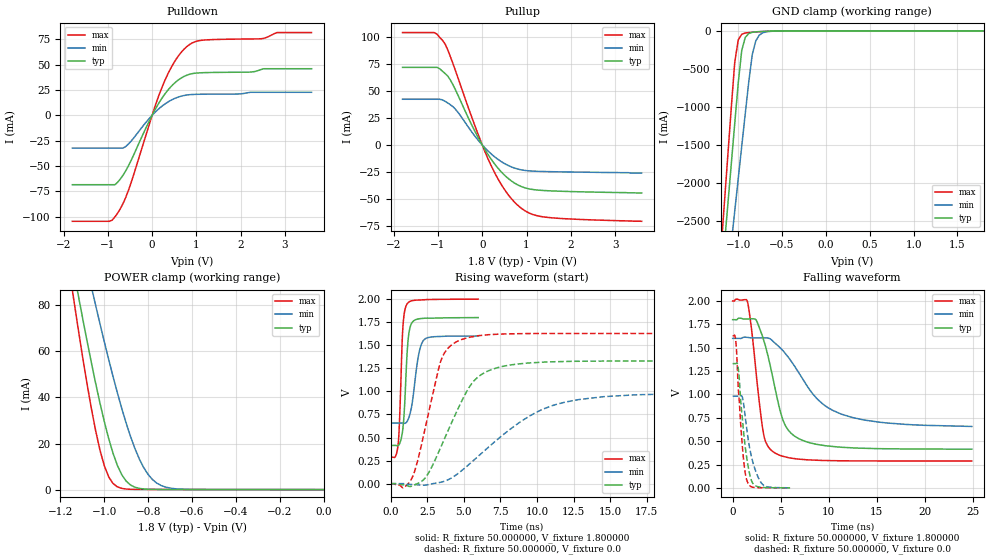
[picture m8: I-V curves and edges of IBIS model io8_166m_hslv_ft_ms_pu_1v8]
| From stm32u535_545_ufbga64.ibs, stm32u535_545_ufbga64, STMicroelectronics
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|   Model io8_166m_hslv_ft_ms_pu_1v8
[Model]  io8_166m_hslv_ft_ms_pu_1v8
Model_type I/O
Polarity   Non-Inverting
Enable   Active-Low
Vinl =   0.540000V
Vinh =   1.260000V
Vmeas =  0.900000V
Cref =   50.000000pF
Rref =   100.000000M
Vref =   0.0V
C_comp   3.358400pF   3.352800pF   3.400400pF
[Temperature Range]   25.000000   0.140000k   -40.000000
[Pullup Reference]   1.800000V   1.600000V   2.000000V
[Pulldown Reference]   0.0V   0.0V   0.0V
[POWER Clamp Reference]   1.800000V   1.600000V   2.000000V
[GND Clamp Reference]   0.0V   0.0V   0.0V
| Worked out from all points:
|   slope of the pulldown table from 0 to 0.27 V, typ, clamps not added: 13.6 ohm
|   slope of the pullup table from 0 to 0.27 V, typ, clamps not added: 15.9 ohm
|   GND clamp passes 1 mA (typ) near -0.51 V on its own axis
|   POWER clamp passes 1 mA (typ) near -0.86 V on its own axis
|   rising waveform, R_fixture 50.000000, V_fixture 1.800000: 20-80 % time 283ps typ, 490ps min, 231ps max; typ from 0.414 V to 1.8 V
|   rising waveform, R_fixture 50.000000, V_fixture 0.0: 20-80 % time 2.38ns typ, 4.83ns min, 1.41ns max; typ from 0 V to 1.33 V
|   falling waveform, R_fixture 50.000000, V_fixture 1.800000: 20-80 % time 1.98ns typ, 4.45ns min, 1.12ns max; typ from 1.8 V to 0.414 V
|   falling waveform, R_fixture 50.000000, V_fixture 0.0: 20-80 % time 798ps typ, 1.05ns min, 633ps max; typ from 1.33 V to 0 V
[Pulldown]
|Voltage   I(typ)   I(min)   I(max)
-1.8V     -68.38mA   -32.32mA   -104.4mA
-960mV    -68.38mA   -32.32mA   -104.4mA
-780mV    -66.08mA   -32.32mA   -96.43mA
-540mV    -50.22mA   -28.51mA   -74.66mA
0V        0A         0A         0A
240mV     18.04mA    9.6mA      29.42mA
480mV     30.68mA    16.02mA    50.95mA
780mV     39.48mA    19.99mA    67.56mA
1.14V     41.99mA    20.78mA    74.01mA
2.46V     45.1mA     22.69mA    75.45mA
2.82V     45.89mA    22.69mA    81.54mA
3.6V      45.89mA    22.69mA    81.54mA
[Pullup]
|Voltage   I(typ)   I(min)   I(max)
-1.8V     71.66mA    42.2mA     103.8mA
-1.08V    71.66mA    42.2mA     103.8mA
-840mV    66.03mA    40.35mA    93.39mA
-720mV    60mA       37.16mA    81.6mA
-600mV    50.51mA    32.72mA    68.08mA
-180mV    13.77mA    8.913mA    19.32mA
180mV     -11.9mA    -7.442mA   -17.26mA
480mV     -26.98mA   -16.65mA   -39.76mA
840mV     -37.65mA   -22.63mA   -57.07mA
1.08V     -40.74mA   -24.01mA   -63.22mA
1.44V     -42.19mA   -24.58mA   -66.73mA
3.6V      -44.3mA    -26mA      -70.5mA
[GND_clamp]
|Voltage   I(typ)   I(min)   I(max)
-1.8V     -9.908A    -9.683A    -9.994A
-1.2V     -3.383A    -4.084A    -2.934A
-1.16V    -2.841A    -3.655A    -2.294A
-1.12V    -2.299A    -3.226A    -1.656A
-1.04V    -1.218A    -2.369A    -414.2mA
-1V       -684.7mA   -1.941A    -119.2mA
-960mV    -257.2mA   -1.514A    -45.66mA
-920mV    -87.03mA   -1.089A    -28.93mA
-840mV    -19.35mA   -312.8mA   -18.97mA
-800mV    -13.55mA   -132.4mA   -15.49mA
-720mV    -8.042mA   -25.67mA   -9.491mA
1.8V      0A         13.64nA    0A
[POWER_clamp]
|Voltage   I(typ)   I(min)   I(max)
-1.8V     470.9mA    433.7mA    554.6mA
-1.14V    95.28mA    122.7mA    82.88mA
-1.12V    85mA       114mA      70.34mA
-1.06V    55.55mA    88.43mA    35.73mA
-1.04V    46.38mA    80.17mA    25.83mA
-1V       29.54mA    64.14mA    10.37mA
-940mV    10.43mA    41.88mA    1.177mA
-900mV    3.66mA     28.79mA    250.5uA
-840mV    527.2uA    13.26mA    96.07uA
-800mV    154.2uA    6.55mA     88.1uA
-740mV    59.7uA     1.741mA    70.27uA
0V        0A         18.18nA    0A
[Ramp]
| variable   typ   min   max
dV/dt_r  0.79757/2.37744n   0.58708/4.82407n   0.97651/1.40841n
dV/dt_f  0.83122/1.97191n   0.56109/4.43761n   1.02743/1.11864n
R_load = 50.000000
[Rising Waveform]
R_fixture= 50.000000
V_fixture= 1.800000
V_fixture_min= 1.600000
V_fixture_max= 2.000000
|time   V(typ)   V(min)   V(max)
0s        414.4mV    657.5mV    287.7mV
516.5ps   412.8mV    657.6mV    425.9mV
612.6ps   432.8mV    657.6mV    690.8mV
828.8ps   582.2mV    656.4mV    1.66V
1.093ns   1.311V     665.6mV    1.938V
1.213ns   1.581V     701mV      1.964V
1.369ns   1.714V     784.1mV    1.978V
1.886ns   1.785V     1.37V      1.99V
2.246ns   1.792V     1.553V     1.993V
5.982ns   1.8V       1.6V       2V
[Rising Waveform]
R_fixture= 50.000000
V_fixture= 0.0
V_fixture_min= 0.0
V_fixture_max= 0.0
|time   V(typ)   V(min)   V(max)
0s        408.8uV    505.3uV    361.6uV
850.9ps   -11.78mV   749.6uV    -45.19mV
1.451ns   -25.98mV   -9.094mV   57.57mV
2.352ns   59.6mV     -15.58mV   593.9mV
3.453ns   403.4mV    16.75mV    1.339V
4.705ns   844.7mV    122.1mV    1.553V
5.656ns   1.108V     250.4mV    1.594V
6.657ns   1.221V     391.3mV    1.614V
11.56ns   1.323V     869.4mV    1.628V
24.92ns   1.33V      980.7mV    1.628V
[Falling Waveform]
R_fixture= 50.000000
V_fixture= 1.800000
V_fixture_min= 1.600000
V_fixture_max= 2.000000
|time   V(typ)   V(min)   V(max)
0s        1.8V       1.6V       2V
1.552ns   1.808V     1.61V      1.989V
2.452ns   1.796V     1.605V     1.224V
3.203ns   1.59V      1.605V     587.4mV
4.304ns   1.122V     1.559V     380.4mV
5.556ns   655.7mV    1.43V      330.3mV
7.658ns   494.4mV    1.107V     301.3mV
9.71ns    450.5mV    873.7mV    292.8mV
12.51ns   428.4mV    752.4mV    289.1mV
24.92ns   414.4mV    657.5mV    287.7mV
[Falling Waveform]
R_fixture= 50.000000
V_fixture= 0.0
V_fixture_min= 0.0
V_fixture_max= 0.0
|time   V(typ)   V(min)   V(max)
0s        1.33V      980.7mV    1.628V
324.3ps   1.33V      980.8mV    1.568V
420.4ps   1.335V     980.8mV    1.438V
552.6ps   1.303V     980.8mV    1.136V
1.093ns   651.1mV    931.3mV    348.9mV
1.297ns   451.3mV    774mV      166.7mV
1.526ns   283.9mV    590.4mV    68.36mV
2.03ns    61.2mV     304.2mV    9.114mV
3.027ns   6.071mV    47.69mV    1.802mV
5.982ns   408.8uV    505.3uV    361.6uV
